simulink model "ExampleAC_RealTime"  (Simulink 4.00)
settings: Solver=FixedStepDiscrete  StartTime=0.0  StopTime=10000.0  FixedStep=0.02  RelTol=1e-3
libraries: AVDSBlockset x1, simulink3 x1

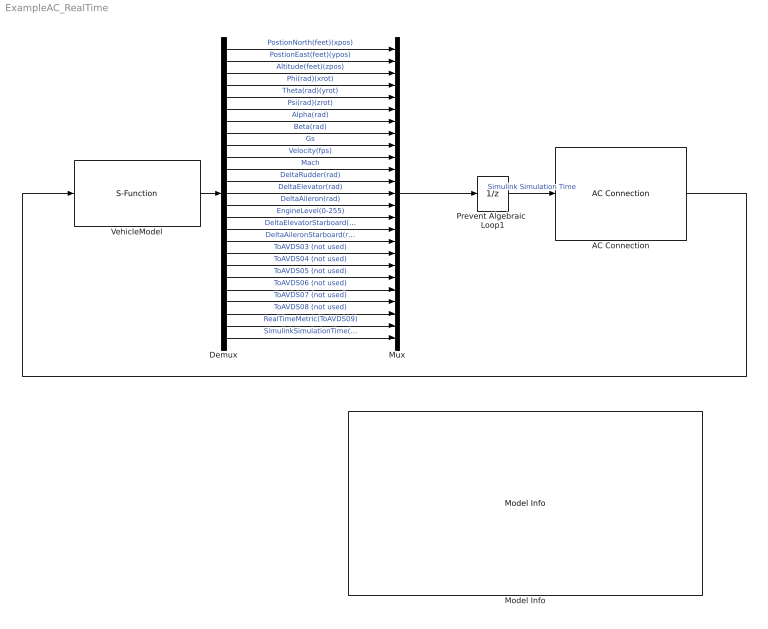
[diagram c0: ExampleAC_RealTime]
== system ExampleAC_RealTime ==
  AC Connection : AVDSBlockset/AC Connection  Description=This block is used to connect Simulink to AVDS through the MATLAB AC model.  RealTime=on
  Demux : Demux  Outputs=25  BusSelectionMode=off
  Model Info : simulink3/Signals & Systems/Model Info  InitialBlockCM=none  BlockCM=none  Frame=off  DisplayStringWithTags=|  HorizontalTextAlignment=Left  LeftAlignmentValue=0.02  SourceBlockDiagram=ExampleAC_RealTime  TagMaxNumber=20
      | Important -  make sure the files in the directory 
      |      "Utilities\MATLABToolbox\Toolbox\RequiredAVDSFiles" are installed
      |       according to the instructions in the file "ReadMe.RequiredAVDSFiles.txt".
      |    To start the simulation:
      |    1) Start AVDS
      |    2) Load the simulation initialization file "MATLAB_AC.sim.ini". From the AVDS 
      |       menu select "File->Simulation Init->Open" and choose the file "MA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
  Mux : Mux  Inputs=25
  Prevent Algebraic  Loop1 : UnitDelay  X0=0  SampleTime=0.02
  VehicleModel : S-Function  FunctionName=AVDS_AC_SimulinkS  PortCounts=[]  SFunctionModules=''
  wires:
  Prevent Algebraic  Loop1/1 -> AC Connection/1  "Simulink Simulation Time"
  VehicleModel/1 -> Demux/1
  Demux/1 -> Mux/1  "PostionNorth(feet)(xpos)"
  Demux/2 -> Mux/2  "PostionEast(feet)(ypos)"
  Demux/3 -> Mux/3  "Altitude(feet)(zpos)"
  Demux/4 -> Mux/4  "Phi(rad)(xrot)"
  Demux/5 -> Mux/5  "Theta(rad)(yrot)"
  Demux/6 -> Mux/6  "Psi(rad)(zrot)"
  Demux/7 -> Mux/7  "Alpha(rad)"
  Demux/8 -> Mux/8  "Beta(rad)"
  Demux/9 -> Mux/9  "Gs"
  Demux/10 -> Mux/10  "Velocity(fps)"
  Demux/11 -> Mux/11  "Mach"
  Demux/12 -> Mux/12  "DeltaRudder(rad)"
  Demux/13 -> Mux/13  "DeltaElevator(rad)"
  Demux/14 -> Mux/14  "DeltaAileron(rad)"
  Demux/16 -> Mux/16  "DeltaElevatorStarboard(rad)(ToAVDS01)"
  Demux/17 -> Mux/17  "DeltaAileronStarboard(rad)(ToAVDS02)"
  Demux/18 -> Mux/18  "ToAVDS03 (not used)"
  Demux/19 -> Mux/19  "ToAVDS04 (not used)"
  Demux/20 -> Mux/20  "ToAVDS05 (not used)"
  Demux/21 -> Mux/21  "ToAVDS06 (not used)"
  Demux/22 -> Mux/22  "ToAVDS07 (not used)"
  Demux/23 -> Mux/23  "ToAVDS08 (not used)"
  Demux/24 -> Mux/24  "RealTimeMetric(ToAVDS09)"
  Demux/25 -> Mux/25  "SimulinkSimulationTime(ToAVDS10)"
  Mux/1 -> Prevent Algebraic  Loop1/1
  Demux/15 -> Mux/15  "EngineLevel(0-255)"
  AC Connection/1 -> VehicleModel/1
